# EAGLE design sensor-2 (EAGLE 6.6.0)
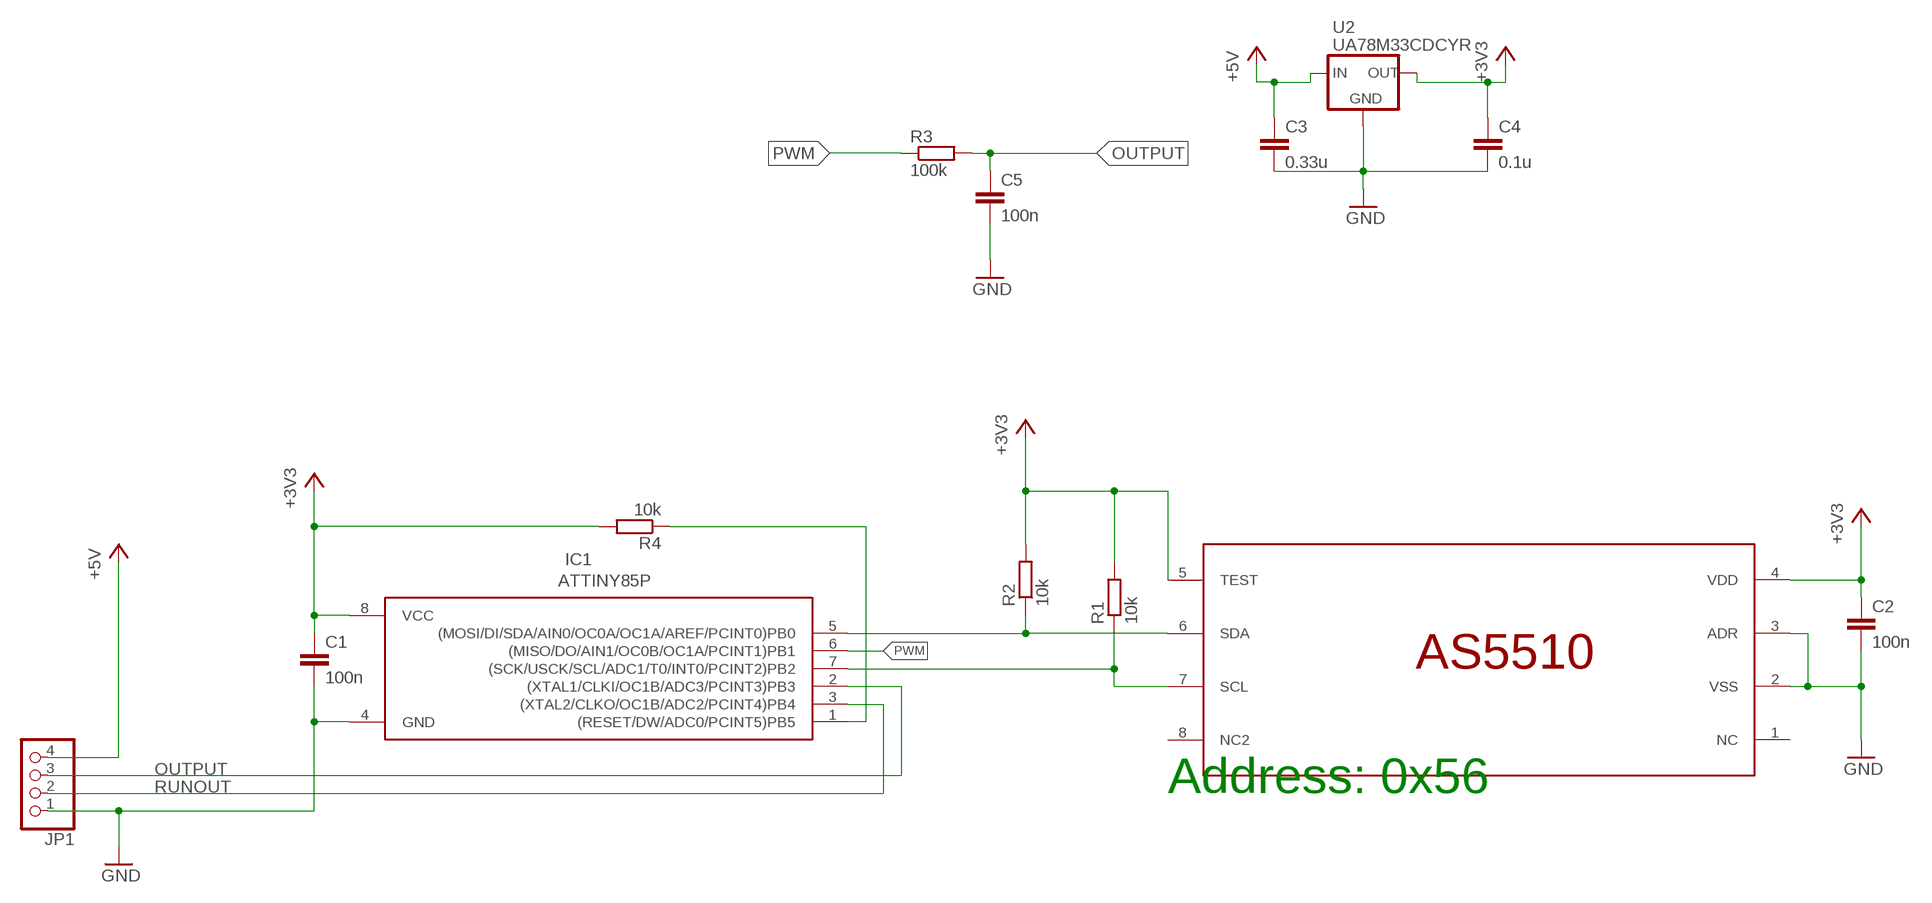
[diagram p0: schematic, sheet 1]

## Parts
C1  100n  C-EUC1206  [C1206]
C2  100n  C-EUC1206  [C1206]
C3  0.33u  C-EUC1206  [C1206]
C4  0.1u  C-EUC1206  [C1206]
C5  100n  C-EUC1206  [C1206]
IC1  ATTINY85P  [DIL08]
JP1  PINHD-1X4  [1X04]
R1  10k  R-EU_R1206  [R1206]
R2  10k  R-EU_R1206  [R1206]
R3  100k  R-EU_R1206  [R1206]
R4  10k  R-EU_R1206  [R1206]
U2  UA78M33CDCYR  [SOT-223]
U$1  AS5510  [SOIC8]

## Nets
+3V3: C1.1 C2.1 C4.1 IC1.8(VCC) R1.2 R2.2 R4.2 U2.3(OUT) U$1.4(VDD) U$1.5(TEST)
+5V: C3.1 JP1.4 U2.1(IN)
GND: C1.2 C2.2 C3.2 C4.2 C5.2 IC1.4(GND) JP1.1 U2.2(GND) U2.4(GND) U$1.2(VSS) U$1.3(ADR)
N$1: IC1.5((MOSI/DI/SDA/AIN0/OC0A/OC1A/AREF/PCINT0)PB0) R2.1 U$1.6(SDA)
N$2: IC1.7((SCK/USCK/SCL/ADC1/T0/INT0/PCINT2)PB2) R1.1 U$1.7(SCL)
N$3: IC1.1((RESET/DW/ADC0/PCINT5)PB5) R4.1
OUTPUT: C5.1 IC1.2((XTAL1/CLKI/OC1B/ADC3/PCINT3)PB3) JP1.3 R3.2
PWM: IC1.6((MISO/DO/AIN1/OC0B/OC1A/PCINT1)PB1) R3.1
RUNOUT: IC1.3((XTAL2/CLKO/OC1B/ADC2/PCINT4)PB4) JP1.2
Unconnected: U$1.1(NC) U$1.8(NC2)

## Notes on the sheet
- Address: 0x56

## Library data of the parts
C1-C5 = resistor:C-EU: CAPACITOR, European symbol
IC1 = atmel-JP:ATTINY85: MICROCONTROLLER 8 Kbytes FLASH 512 bytes EEPROM 512 bytes RAM 4-channel 10 bit ADC USI
JP1 = pinhead:PINHD-1X4: PIN HEADER
R1-R4 = resistor:R-EU_: RESISTOR, European symbol
U2 = TI:UA78M33
U$1 = as5510:AS5510: The AS5510 is a Linear Hall Sensor with 10 bit resolution and I²C interface.

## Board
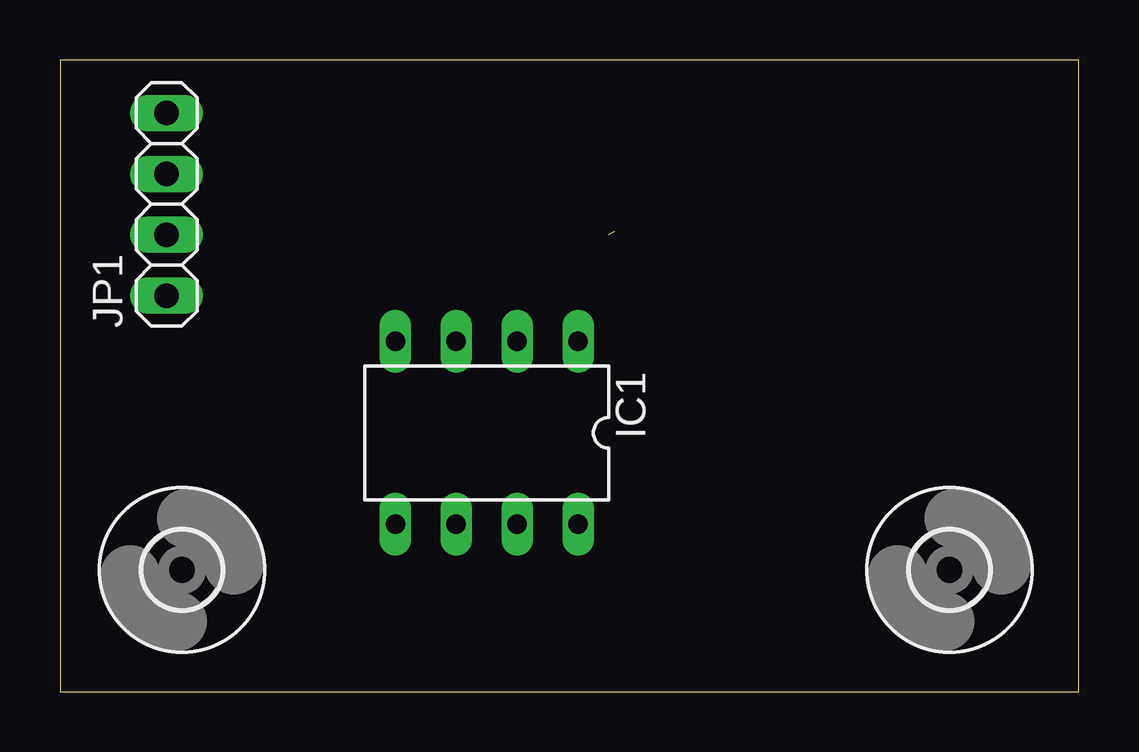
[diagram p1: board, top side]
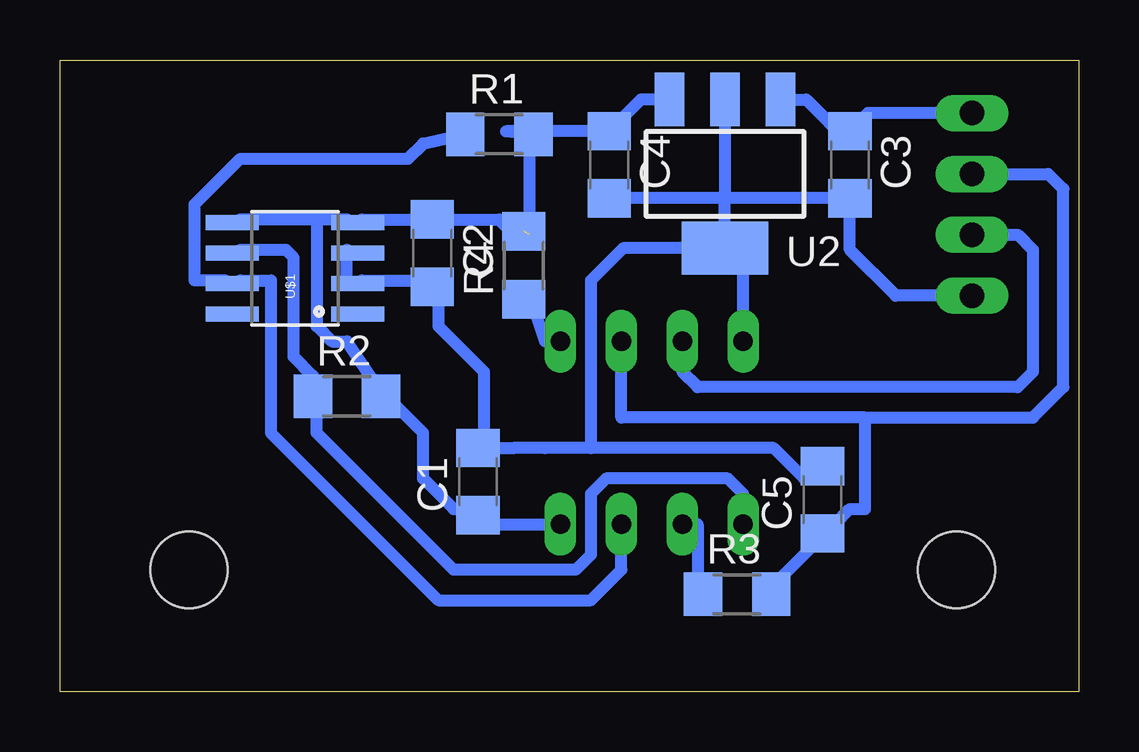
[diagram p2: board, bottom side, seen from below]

Size 42.44 x 26.34 mm. Coordinates in mm from the lower left corner, seen from the top.
Outline: 0,0 42.44,0 42.44,26.34 0,26.34 0,0
Copper layers (1*16): Top 0.035mm / dielectric 1.5mm / Bottom 0.035mm
Design rules "Pasch20": minimum track width 20mil, minimum drill 24mil, track to track 8mil, track to pad 8mil, pad to pad 8mil, via to via 8mil, smd to smd 8mil, copper to edge 5mil, drill to drill 8mil, minimum pad ring 10mil, minimum via ring 8mil, stop-mask expansion 0mil, vias tented up to drill 0mil, thermal gap 10mil

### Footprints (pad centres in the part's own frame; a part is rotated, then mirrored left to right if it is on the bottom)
C1206 = smd 1.6 x 1.8: 1 -1.4,0; 2 1.4,0
DIL08 = drill 0.813 long: 1 -3.81,-3.81; 2 -1.27,-3.81; 3 1.27,-3.81; 4 3.81,-3.81; 5 3.81,3.81; 6 1.27,3.81; 7 -1.27,3.81; 8 -3.81,3.81
1X04 = drill 1.016 long: 1 -3.81,0; 2 -1.27,0; 3 1.27,0; 4 3.81,0
R1206 = smd 1.6 x 1.803: 1 -1.422,0; 2 1.422,0
SOT-223 = smd 1.219 x 2.235: 1 -2.311,-3.099; 2 0,-3.099; 3 2.311,-3.099 | smd 3.6 x 2.2: 4 0,3.099
SOIC8 = smd 0.61 x 2.21: 1 -1.905,-2.616; 2 -0.635,-2.616; 3 0.635,-2.616; 4 1.905,-2.616; 5 1.905,2.616; 6 0.635,2.616; 7 -0.635,2.616; 8 -1.905,2.616
3,2 = hole 3.2: 0,0

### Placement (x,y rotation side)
C1  25.02,8.76 90 bottom
C2  26.92,18.29 270 bottom
C3  9.53,21.97 270 bottom
C4  19.56,21.97 270 bottom
C5  10.67,8 90 bottom
IC1  17.78,10.8 180 top
JP1  4.45,20.32 90 top
R1  24.13,23.24 0 bottom
R2  30.48,12.32 0 bottom
R3  14.22,4.06 0 bottom
R4  23.11,17.78 90 bottom
U2  14.73,21.59 180 bottom
U$1  32.64,17.65 90 bottom
U$2  [3,2]  5.08,5.08 0 top
U$3  [3,2]  37.06,5.08 0 top

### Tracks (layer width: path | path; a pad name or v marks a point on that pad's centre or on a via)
+3V3  (1 unrouted)
  Bottom 0.508: 31.75,19.69 30.48,19.69 U$1.4 29.84,19.69 27.3,19.69 C2.1 26.67,19.69 24.13,19.69 23.5,19.05 22.86,19.05 22.86,22.86 R1.2 23.85,23.37 C4.1 18.24,24.69 U2.3 | 31.75,19.69 34.92,19.69 U$1.5 | 31.75,19.69 31.75,15.24 31.11,14.61 30.48,14.61 29.21,12.7 28.83,12.32 R2.2 28.57,12.06 27.3,10.8 27.3,8.89 26.04,7.62 25.14,7.36 C1.1 25.02,7.24 24.77,6.98 IC1.8
+5V
  Bottom 0.508: U2.1 11.35,24.69 9.53,22.86 C3.1 8.77,24.13 JP1.4
GND
  Bottom 0.508: U$1.3 30.48,18.41 30.48,17.14 U$1.2 29.84,17.14 27.3,17.14 C2.2 26.67,16.51 26.67,15.24 24.77,13.34 24.77,10.8 25.02,10.54 C1.2 23.5,10.16 22.23,10.16 20.32,10.16 | 20.32,10.16 12.7,10.16 11.43,8.89 10.79,8.89 C5.2 | 14.61,20.57 C3.2 9.53,18.41 7.62,16.51 JP1.1 | 14.61,20.57 C4.2 | U2.4 14.73,20.44 14.61,20.57 | U2.2 14.73,20.7 14.61,20.57 | U2.4 18.97,18.49 20.32,17.14 20.32,10.16 | IC1.4 13.97,17.73 U2.4
N$1
  Bottom 0.508: U$1.6 34.92,18.41 33.02,18.41 32.7,18.1 32.7,13.97 31.9,13.17 R2.1 31.75,12.06 31.75,10.8 26.04,5.08 20.95,5.08 20.32,5.71 20.32,8.25 19.68,8.89 14.61,8.89 13.97,8.25 IC1.5
N$2
  Bottom 0.508: R1.1 27.3,22.86 27.94,22.22 34.92,22.22 36.83,20.32 36.83,17.14 35.56,17.14 U$1.7 34.92,17.14 33.66,17.14 33.66,10.8 26.67,3.81 20.32,3.81 19.05,5.08 IC1.7
N$3
  Bottom 0.508: IC1.1 22.23,14.61 22.86,16.51 R4.1
OUTPUT
  Bottom 0.508: R3.2 12.7,4.45 10.79,6.35 C5.1 10.16,6.98 9.53,7.62 8.89,7.62 8.89,11.43 | IC1.2 19.05,11.43 8.89,11.43 | 8.89,11.43 1.91,11.43 0.64,12.7 0.64,20.95 1.27,21.59 JP1.3
PWM
  Bottom 0.508: IC1.6 15.88,6.98 15.88,4.45 R3.1
RUNOUT
  Bottom 0.508: JP1.2 2.54,19.05 1.91,18.41 1.91,13.34 2.54,12.7 15.88,12.7 16.51,13.34 IC1.3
